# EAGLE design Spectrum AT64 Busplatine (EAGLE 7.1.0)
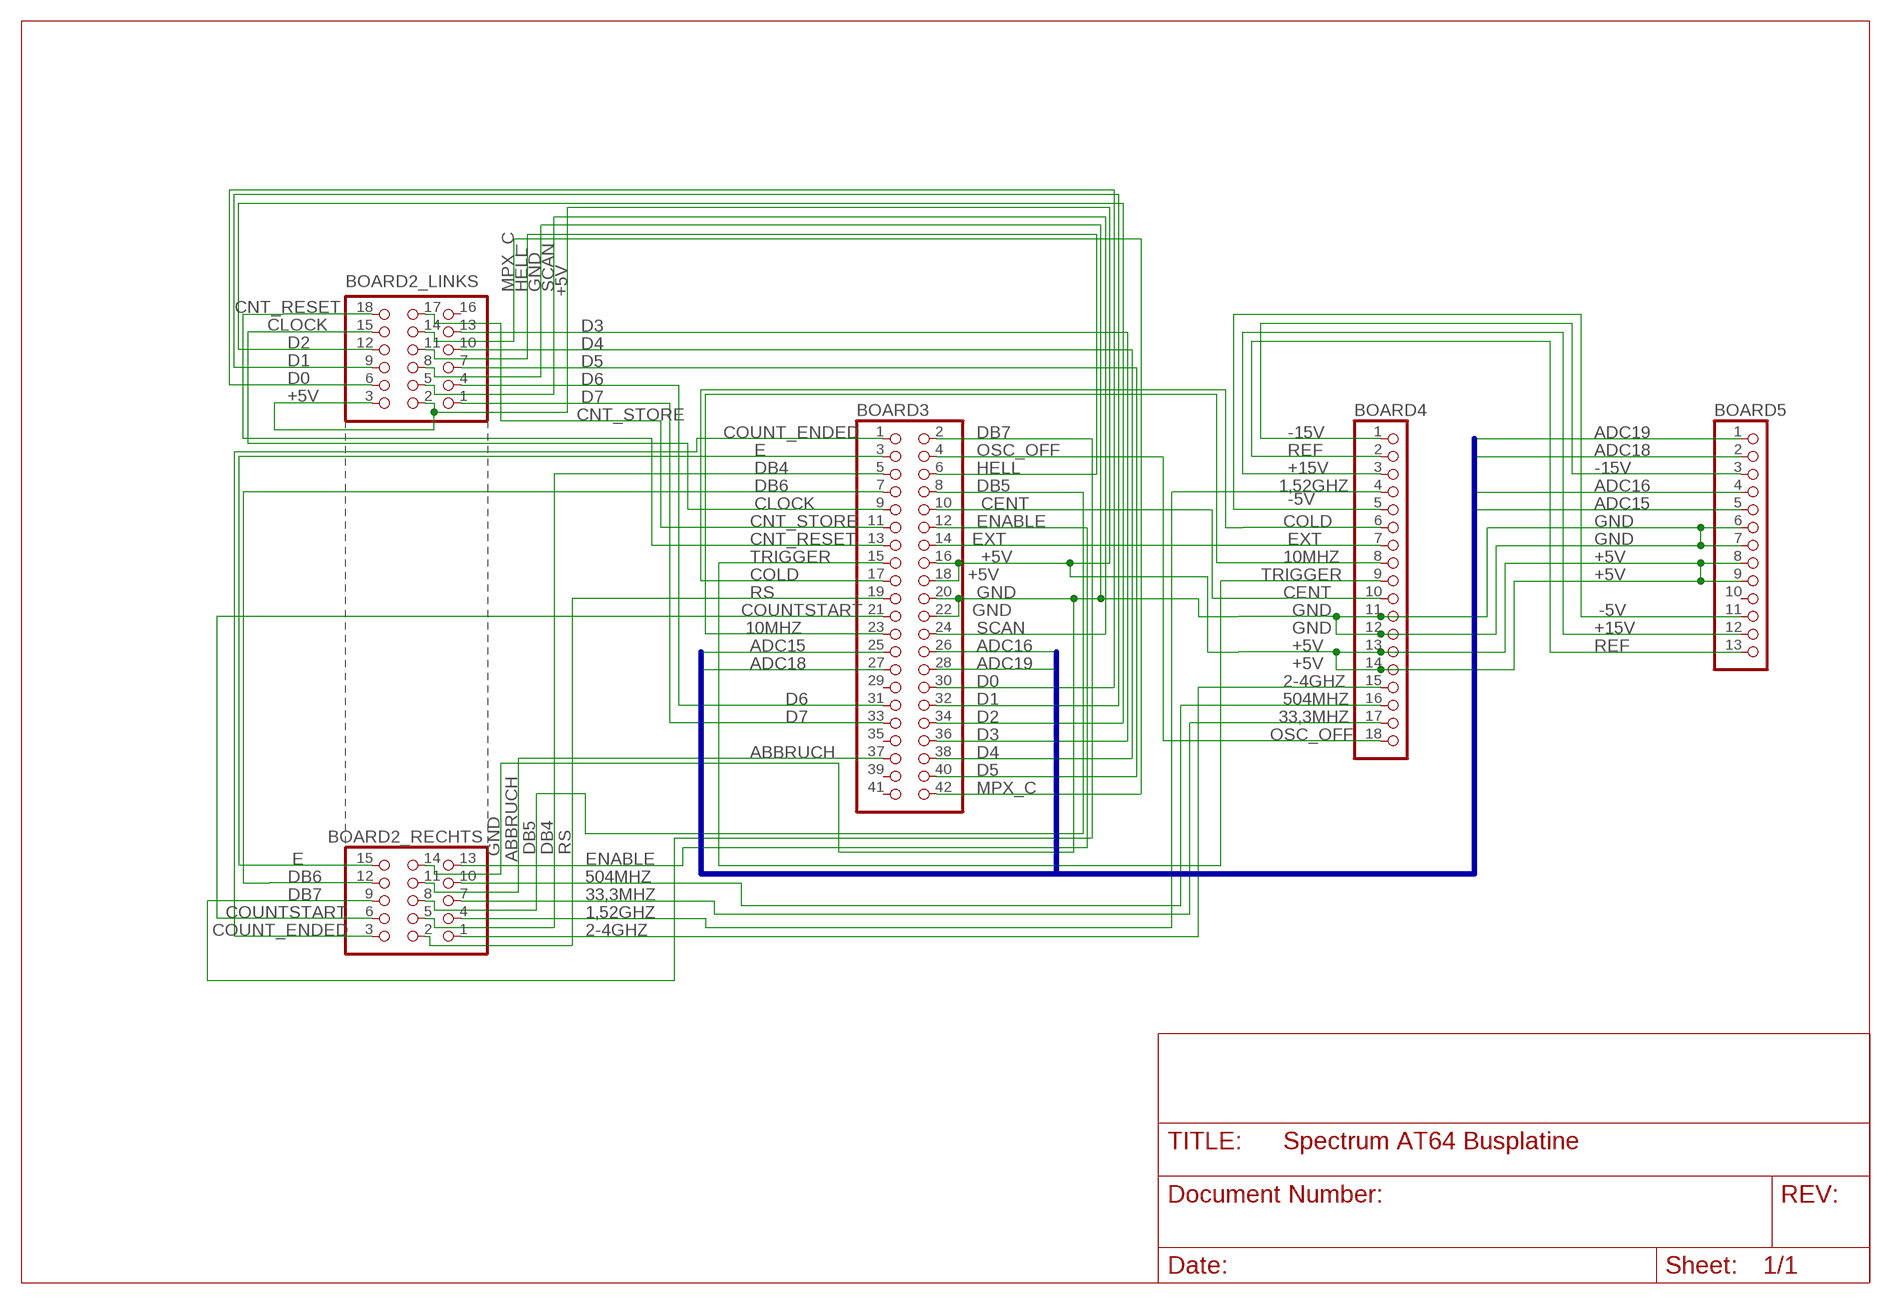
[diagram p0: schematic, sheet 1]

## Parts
BOARD2_LINKS  6X3/90  [6X3/90]
BOARD2_RECHTS  5X3/90  [5X3/90]
BOARD3  PINHD-2X21_2.54  [2X21]
BOARD4  PINHD-1X18  [1X18]
BOARD5  PINHD-1X13_2.54  [1X13]

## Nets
1,52GHZ: BOARD2_RECHTS.4 BOARD4.4
2-4GHZ: BOARD2_RECHTS.1 BOARD4.15
10MHZ: BOARD3.23 BOARD4.8
33,3MHZ: BOARD2_RECHTS.7 BOARD4.17
504MHZ: BOARD2_RECHTS.10 BOARD4.16
+5V: BOARD2_LINKS.2 BOARD2_LINKS.3 BOARD3.16 BOARD3.18 BOARD4.13 BOARD4.14 BOARD5.8 BOARD5.9
+15V: BOARD4.3 BOARD5.12
-5V: BOARD4.5 BOARD5.11
-15V: BOARD4.1 BOARD5.3
ABBRUCH: BOARD2_RECHTS.11 BOARD3.37
ADC15: BOARD3.25 BOARD5.5
ADC16: BOARD3.26 BOARD5.4
ADC18: BOARD3.27 BOARD5.2
ADC19: BOARD3.28 BOARD5.1
CENT: BOARD3.10 BOARD4.10
CLOCK: BOARD2_LINKS.15 BOARD3.9
CNT_RESET: BOARD2_LINKS.18 BOARD3.13
CNT_STORE: BOARD2_LINKS.17 BOARD3.11
COLD: BOARD3.17 BOARD4.6
COUNT_ENDED: BOARD2_RECHTS.3 BOARD3.1
COUNTSTART: BOARD2_RECHTS.6 BOARD3.21
D0: BOARD2_LINKS.6 BOARD3.30
D1: BOARD2_LINKS.9 BOARD3.32
D2: BOARD2_LINKS.12 BOARD3.34
D3: BOARD2_LINKS.13 BOARD3.36
D4: BOARD2_LINKS.10 BOARD3.38
D5: BOARD2_LINKS.7 BOARD3.40
D6: BOARD2_LINKS.4 BOARD3.31
D7: BOARD2_LINKS.1 BOARD3.33
DB4: BOARD2_RECHTS.5 BOARD3.5
DB5: BOARD2_RECHTS.8 BOARD3.8
DB6: BOARD2_RECHTS.12 BOARD3.7
DB7: BOARD2_RECHTS.9 BOARD3.2
E: BOARD2_RECHTS.15 BOARD3.3
ENABLE: BOARD2_RECHTS.13 BOARD3.12
EXT: BOARD3.14 BOARD4.7
GND: BOARD2_LINKS.8 BOARD2_RECHTS.14 BOARD3.20 BOARD3.22 BOARD4.11 BOARD4.12 BOARD5.6 BOARD5.7
HELL: BOARD2_LINKS.11 BOARD3.6
MPX_C: BOARD2_LINKS.14 BOARD3.42
OSC_OFF: BOARD3.4 BOARD4.18
REF: BOARD4.2 BOARD5.13
RS: BOARD2_RECHTS.2 BOARD3.19
SCAN: BOARD2_LINKS.5 BOARD3.24
TRIGGER: BOARD3.15 BOARD4.9
Unconnected: BOARD2_LINKS.16 BOARD3.29 BOARD3.35 BOARD3.39 BOARD3.41 BOARD5.10

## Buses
ADC15,ADC16,ADC18,ADC19

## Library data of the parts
BOARD2_LINKS = 1Eigene:6X3/90
BOARD2_RECHTS = 1Eigene:5X3/90
BOARD3 = pinhead-2:PINHD-2X21: PIN HEADER
BOARD4 = pinhead:PINHD-1X18: PIN HEADER
BOARD5 = pinhead-2:PINHD-1X13: PIN HEADER

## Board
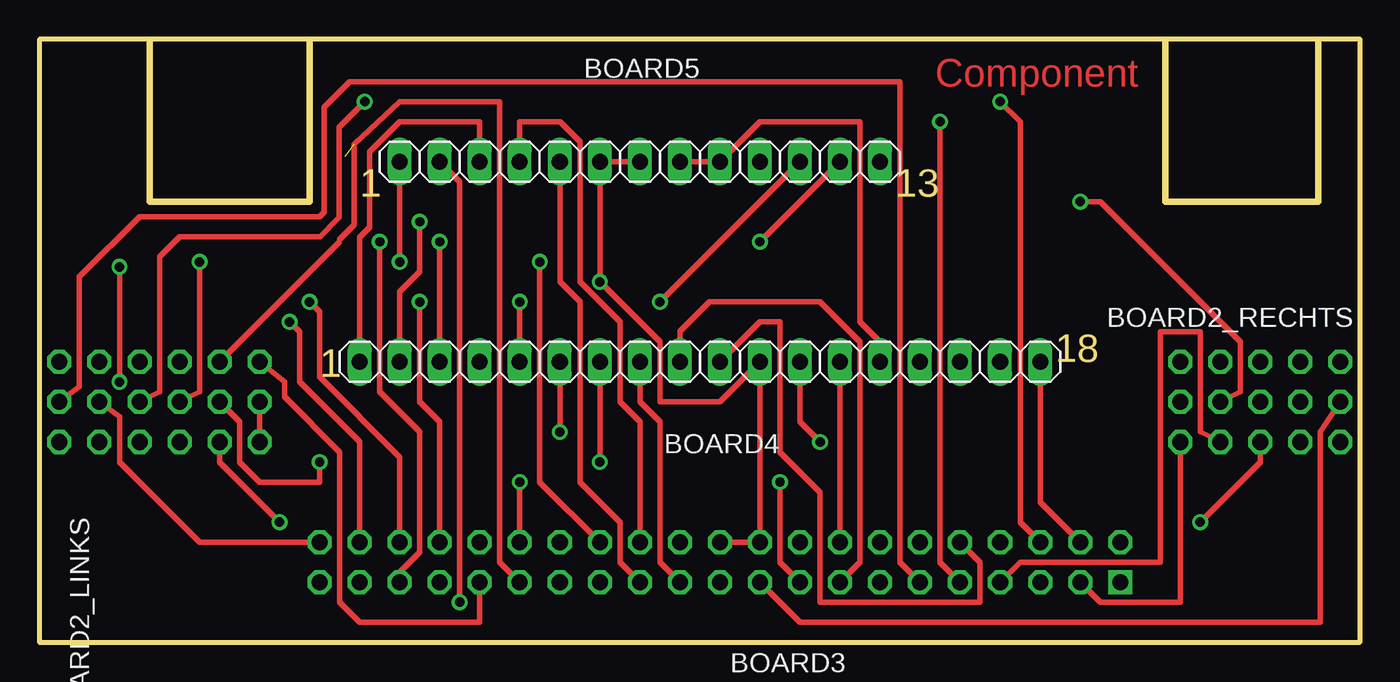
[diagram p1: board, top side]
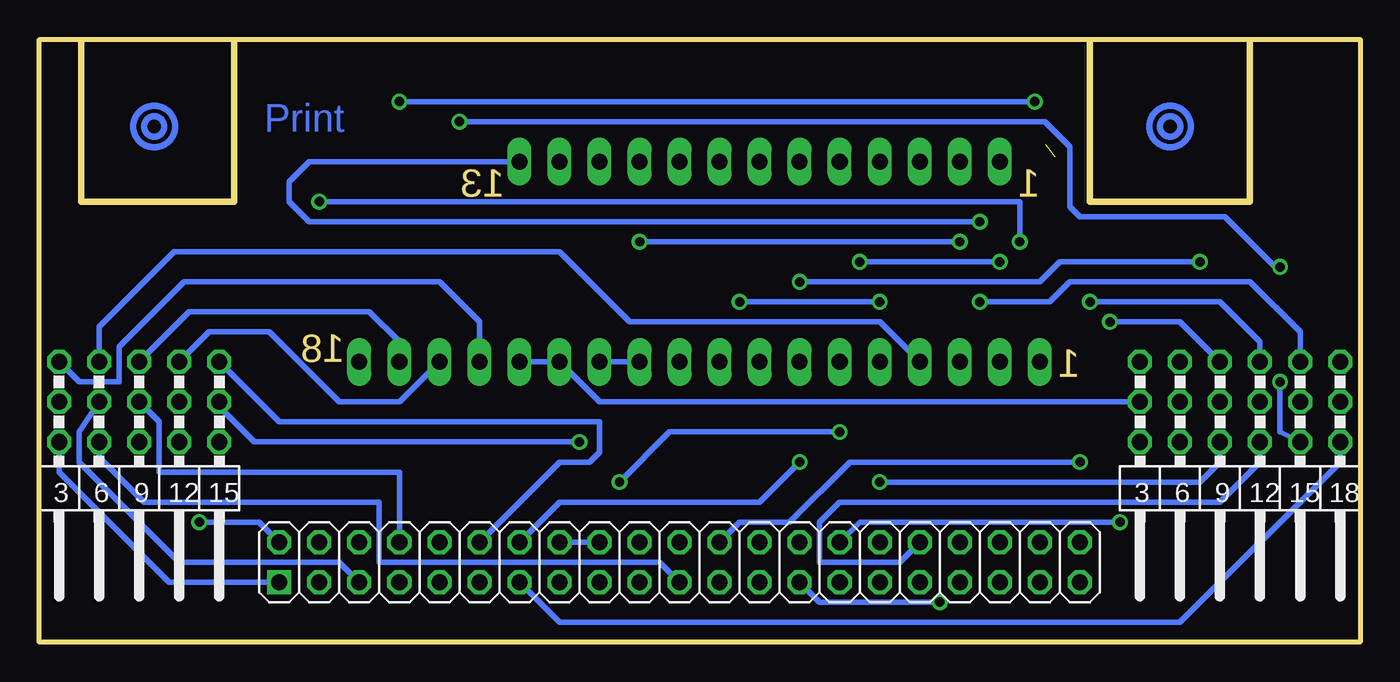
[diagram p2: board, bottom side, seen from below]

Size 83.8 x 38.23 mm. Coordinates in mm from the lower left corner, seen from the top.
Outline: 6.99,38.1 6.99,27.94 17.14,27.94 17.14,38.1
Outline: 71.44,38.1 71.44,27.94 81.13,27.94 81.13,38.1
Outline: 0,0 83.8,0 83.8,38.23 0,38.23 0,0
Copper layers (1*16): Top 0.035mm / dielectric 1.5mm / Bottom 0.035mm
Design rules "default *": minimum track width 0.35mm, minimum drill 0.0152mm, track to track 0.2mm, track to pad 0.2mm, pad to pad 0.2mm, via to via 0.2mm, smd to smd 0.2mm, copper to edge 0.4mm, drill to drill 8mil, minimum pad ring 10mil, minimum via ring 8mil, stop-mask expansion 4mil, vias tented up to drill 0mil, thermal gap 10mil

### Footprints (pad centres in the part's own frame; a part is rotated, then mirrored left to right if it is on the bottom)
6X3/90 = drill 1.016 octagon: 1 6.35,-7.62; 2 6.35,-5.08; 3 6.35,-2.54; 4 3.81,-7.62; 5 3.81,-5.08; 6 3.81,-2.54; 7 1.27,-7.62; 8 1.27,-5.08; 9 1.27,-2.54; 10 -1.27,-7.62; 11 -1.27,-5.08; 12 -1.27,-2.54; 13 -3.81,-7.62; 14 -3.81,-5.08; 15 -3.81,-2.54; 16 -6.35,-7.62; 17 -6.35,-5.08; 18 -6.35,-2.54
5X3/90 = drill 1.016 octagon: 1 5.08,-7.62; 2 5.08,-5.08; 3 5.08,-2.54; 4 2.54,-7.62; 5 2.54,-5.08; 6 2.54,-2.54; 7 0,-7.62; 8 0,-5.08; 9 0,-2.54; 10 -2.54,-7.62; 11 -2.54,-5.08; 12 -2.54,-2.54; 13 -5.08,-7.62; 14 -5.08,-5.08; 15 -5.08,-2.54
2X21 = drill 1.016 square: 1 -24.13,-1.27 | drill 1.016 octagon: 2 -24.13,1.27; 3 -21.59,-1.27; 4 -21.59,1.27; 5 -19.05,-1.27; 6 -19.05,1.27; 7 -16.51,-1.27; 8 -16.51,1.27; 9 -13.97,-1.27; 10 -13.97,1.27; 11 -11.43,-1.27; 12 -11.43,1.27; 13 -8.89,-1.27; 14 -8.89,1.27; 15 -6.35,-1.27; 16 -6.35,1.27; 17 -3.81,-1.27; 18 -3.81,1.27; 19 -1.27,-1.27; 20 -1.27,1.27; 21 1.27,-1.27; 22 1.27,1.27; 23 3.81,-1.27; 24 3.81,1.27; 25 6.35,-1.27; 26 6.35,1.27; 27 8.89,-1.27; 28 8.89,1.27; 29 11.43,-1.27; 30 11.43,1.27; 31 13.97,-1.27; 32 13.97,1.27; 33 16.51,-1.27; 34 16.51,1.27; 35 19.05,-1.27; 36 19.05,1.27; 37 21.59,-1.27; 38 21.59,1.27; 39 24.13,-1.27; 40 24.13,1.27; 41 26.67,-1.27; 42 26.67,1.27
1X18 = drill 1.016 long: 1 -21.59,0; 2 -19.05,0; 3 -16.51,0; 4 -13.97,0; 5 -11.43,0; 6 -8.89,0; 7 -6.35,0; 8 -3.81,0; 9 -1.27,0; 10 1.27,0; 11 3.81,0; 12 6.35,0; 13 8.89,0; 14 11.43,0; 15 13.97,0; 16 16.51,0; 17 19.05,0; 18 21.59,0
1X13 = drill 1.016 long: 1 -15.24,0; 2 -12.7,0; 3 -10.16,0; 4 -7.62,0; 5 -5.08,0; 6 -2.54,0; 7 0,0; 8 2.54,0; 9 5.08,0; 10 7.62,0; 11 10.16,0; 12 12.7,0; 13 15.24,0

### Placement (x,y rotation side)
BOARD2_LINKS  7.62,10.16 180 bottom
BOARD2_RECHTS  77.47,10.16 180 bottom
BOARD3  44.45,5.08 0 bottom
BOARD4  41.91,17.78 0 top
BOARD5  38.1,30.48 0 top

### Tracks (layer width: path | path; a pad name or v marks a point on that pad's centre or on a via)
1,52GHZ
  Bottom 0.35: BOARD4.4 30.48,20.32 46.35,20.32 50.8,24.77 75.25,24.77 80.01,20 BOARD2_RECHTS.4
2-4GHZ
  Bottom 0.35: BOARD4.15 55.88,20.32 58.42,22.86 74.61,22.86 78.74,18.73 78.74,16.51 81.28,16.51 BOARD2_RECHTS.1
10MHZ
  Top 0.35: BOARD3.23 39.37,5.08 39.37,13.97 38.1,15.24 BOARD4.8
33,3MHZ
  Bottom 0.35: BOARD4.17 60.96,19.05 62.87,20.95 74.3,20.95 BOARD2_RECHTS.7
504MHZ
  Bottom 0.35: BOARD2_RECHTS.10 73.03,19.68 69.22,19.68 64.77,15.24 60.96,15.24 BOARD4.16
+5V
  Top 0.35: BOARD5.8 BOARD5.9 45.72,33.02 52.07,33.02 52.07,20.32 53.34,19.05 BOARD4.14 | BOARD2_LINKS.3 BOARD2_LINKS.2 | BOARD4.13 BOARD3.16
  Bottom 0.35: BOARD3.16 BOARD3.18 | BOARD4.14 BOARD4.13 48.26,15.24 BOARD2_LINKS.2
+15V  (via drill 0.6 pad 0.8)
  Top 0.35: BOARD4.3 v25.4,25.4 | v45.72,25.4 BOARD5.12
  Bottom 0.35: v25.4,25.4 v45.72,25.4
-5V  (via drill 0.6 pad 0.8)
  Top 0.35: BOARD4.5 v30.48,21.59 | v39.37,21.59 BOARD5.11
  Bottom 0.35: v30.48,21.59 v39.37,21.59
-15V
  Top 0.35: BOARD5.3 27.94,33.02 22.86,33.02 20.95,31.11 20.95,26.33 20.32,25.69 BOARD4.1
ABBRUCH  (via drill 0.6 pad 0.8)
  Top 0.35: v66.04,27.94 67.31,27.94 68.9,26.35 76.2,19.05 76.2,15.88 BOARD2_RECHTS.11 | BOARD3.37 22.86,4.45 24.13,5.71 24.13,13.34 21.59,15.88 v21.59,25.4
  Bottom 0.35: v66.04,27.94 21.59,27.94 v21.59,25.4
ADC15
  Top 0.35: BOARD3.25 36.83,5.08 36.83,7.62 34.29,10.16 34.29,21.59 33.02,22.86 BOARD5.5
ADC16
  Top 0.35: BOARD3.26 38.1,13.97 36.83,15.24 36.83,20.32 34.29,22.86 34.29,31.75 33.02,33.02 30.48,33.02 BOARD5.4
ADC18  (via drill 0.6 pad 0.8)
  Top 0.35: v26.67,2.54 26.67,29.21 BOARD5.2
  Bottom 0.35: BOARD3.27 34.29,2.54 v26.67,2.54
ADC19  (via drill 0.6 pad 0.8)
  Top 0.35: BOARD3.28 31.75,10.16 v31.75,24.13 | v22.86,24.13 BOARD5.1
  Bottom 0.35: v31.75,24.13 v22.86,24.13
CENT
  Top 0.35: BOARD4.10 45.72,20.32 46.99,20.32 46.99,12.06 49.53,9.53 49.53,2.54 59.69,2.54 59.69,5.08 BOARD3.10
CLOCK  (via drill 0.6 pad 0.8)
  Top 0.35: v5.08,16.51 v5.08,23.81 | v57.15,33.02 57.15,5.08 BOARD3.9
  Bottom 0.35: BOARD2_LINKS.15 5.08,13.34 v5.08,16.51 | v5.08,23.81 5.4,23.81 8.57,26.99 17.78,26.99 18.41,27.62 18.41,31.43 20,33.02 v57.15,33.02
CNT_RESET
  Bottom 0.35: BOARD3.13 50.8,1.27 11.43,1.27 1.27,11.43 BOARD2_LINKS.18
CNT_STORE
  Top 0.35: BOARD2_LINKS.17 2.54,16.19 2.54,23.18 6.35,26.99 17.78,26.99 18.07,27.28 18.07,33.95 19.68,35.56 54.61,35.56 54.61,5.08 BOARD3.11
COLD  (via drill 0.6 pad 0.8)
  Top 0.35: v33.02,13.34 BOARD4.6 | v46.99,10.16 46.99,5.08 BOARD3.17
  Bottom 0.35: v33.02,13.34 43.81,13.34 v46.99,10.16
COUNT_ENDED
  Bottom 0.35: BOARD3.1 75.56,3.81 82.55,10.79 BOARD2_RECHTS.3
COUNTSTART
  Bottom 0.35: BOARD3.21 44.45,5.08 62.23,5.08 62.23,8.89 77.15,8.89 80.01,11.75 BOARD2_RECHTS.6
D0  (via drill 0.6 pad 0.8)
  Top 0.35: v15.24,7.62 11.43,11.43 BOARD2_LINKS.6
  Bottom 0.35: v15.24,7.62 31.75,7.62 BOARD3.30
D1  (via drill 0.6 pad 0.8)
  Top 0.35: v30.48,10.16 BOARD3.32
  Bottom 0.35: v30.48,10.16 10.16,10.16 8.89,11.43 BOARD2_LINKS.9
D2
  Bottom 0.35: BOARD3.34 29.21,5.08 34.29,5.08 34.29,7.62 33.02,8.89 8.89,8.89 6.35,11.43 BOARD2_LINKS.12
D3  (via drill 0.6 pad 0.8)
  Top 0.35: v24.13,21.59 24.13,15.24 25.4,13.97 BOARD3.36
  Bottom 0.35: v24.13,21.59 19.68,21.59 18.41,22.86 6.99,22.86 3.81,19.68 BOARD2_LINKS.13
D4  (via drill 0.6 pad 0.8)
  Top 0.35: BOARD3.38 22.86,11.75 17.78,16.83 17.78,20.95 v17.14,21.59
  Bottom 0.35: v17.14,21.59 8.89,21.59 6.35,19.05 BOARD2_LINKS.10
D5  (via drill 0.6 pad 0.8)
  Top 0.35: BOARD3.40 20.32,12.7 16.51,16.51 16.51,19.68 v15.88,20.32
  Bottom 0.35: BOARD2_LINKS.7 11.43,20.32 v15.88,20.32
D6  (1 unrouted)
  Top 0.35: BOARD2_LINKS.4 19.02,25.38 19.05,25.55 19.98,26.47 19.98,31.58 22.86,34.29 29.21,34.29 29.21,5.08 BOARD3.31
D7
  Top 0.35: BOARD3.33 27.94,1.27 20.32,1.27 19.05,2.54 19.05,12.06 15.56,15.56 15.56,16.51 BOARD2_LINKS.1
DB4
  Bottom 0.35: BOARD3.5 64.77,5.08 74.93,5.08 81.28,11.43 81.28,13.34 BOARD2_RECHTS.5
DB5
  Bottom 0.35: BOARD3.8 60.96,10.79 76.2,10.79 76.2,13.97 BOARD2_RECHTS.8
DB6
  Top 0.35: BOARD3.7 62.23,5.08 71.12,5.08 71.12,19.68 73.66,19.68 73.66,13.34 BOARD2_RECHTS.12
DB7  (via drill 0.6 pad 0.8)
  Top 0.35: v73.66,7.62 77.47,11.43 BOARD2_RECHTS.9
  Bottom 0.35: BOARD3.2 69.85,7.62 v73.66,7.62
E
  Top 0.35: BOARD3.3 67.31,2.54 72.39,2.54 BOARD2_RECHTS.15
ENABLE
  Bottom 0.35: BOARD3.12 50.8,11.43 48.9,11.43 48.26,12.06 48.26,13.97 68.58,13.97 BOARD2_RECHTS.13
EXT  (via drill 0.6 pad 0.8)
  Top 0.35: v35.56,11.43 BOARD4.7
  Bottom 0.35: v35.56,11.43 38.1,8.89 50.8,8.89 BOARD3.14
GND  (via drill 0.6 pad 0.8)
  Top 0.35: BOARD3.22 BOARD3.20 BOARD4.11 43.18,15.24 39.37,15.24 39.37,19.05 v35.56,22.86 BOARD5.6 BOARD5.7 | v49.53,12.7 48.26,13.97 BOARD4.12 | BOARD2_LINKS.8 10.16,15.88 v10.16,24.13
  Bottom 0.35: BOARD4.11 BOARD4.12 | v49.53,12.7 70.17,12.7 72.39,14.92 BOARD2_RECHTS.14 | v10.16,24.13 19.05,24.13 20.32,22.86 v35.56,22.86
HELL  (via drill 0.6 pad 0.8)
  Top 0.35: BOARD2_LINKS.11 7.62,15.88 7.62,24.45 8.89,25.72 17.8,25.72 19.02,26.96 19.02,32.68 v20.64,34.29 | v60.96,34.29 62.23,33.02 62.23,7.62 BOARD3.6
  Bottom 0.35: v20.64,34.29 v60.96,34.29
MPX_C
  Top 0.35: BOARD2_LINKS.14 5.08,14.29 5.08,11.43 10.16,6.35 BOARD3.42
OSC_OFF
  Top 0.35: BOARD3.4 63.5,8.89 BOARD4.18
REF  (via drill 0.6 pad 0.8)
  Top 0.35: BOARD4.2 22.86,22.23 24.13,23.5 v24.13,26.67
  Bottom 0.35: BOARD5.13 66.67,30.48 67.94,29.21 67.94,27.94 66.67,26.67 v24.13,26.67
RS
  Top 0.35: BOARD3.19 48.26,1.27 81.28,1.27 81.28,13.34 BOARD2_RECHTS.2
SCAN  (via drill 0.6 pad 0.8)
  Top 0.35: BOARD2_LINKS.5 12.7,13.97 12.7,11.43 13.97,10.16 17.78,10.16 v17.78,11.43
  Bottom 0.35: v17.78,11.43 32.38,11.43 36.2,7.62 39.37,7.62 BOARD3.24
TRIGGER
  Top 0.35: BOARD3.15 52.07,5.08 52.07,19.05 49.52,21.6 42.52,21.6 40.64,19.72 BOARD4.9
(copper drawn outside any net)
  shapes: Bottom circle x4

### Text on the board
Top: Component
Bottom: Print
Dimension: 1 | 13 | 18 | 1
